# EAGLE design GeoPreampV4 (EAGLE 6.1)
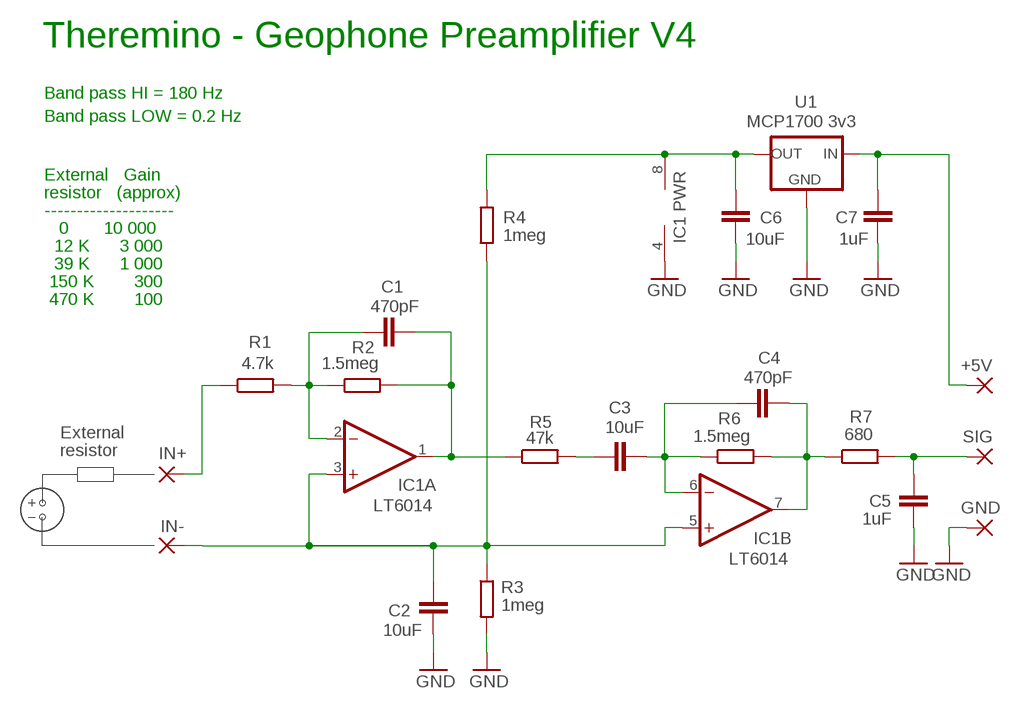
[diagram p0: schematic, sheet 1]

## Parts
+5V  WIREPADSMD1,27-2,54  [SMD1,27-2,54]
C1  470pF  C-EUC0805  [C0805]
C2  10uF  C-EUC0805  [C0805]
C3  10uF  C-EUC0805  [C0805]
C4  470pF  C-EUC0805  [C0805]
C5  1uF  C-EUC0805  [C0805]
C6  10uF  C-EUC0805  [C0805]
C7  1uF  C-EUC0805  [C0805]
GND  WIREPADSMD1,27-2,54  [SMD1,27-2,54]
IC1  LT6014  LMC6482D  [SOIC08_S]
IN+  WIREPADSMD1,27-2,54  [SMD1,27-2,54]
IN-  WIREPADSMD1,27-2,54  [SMD1,27-2,54]
R1  4.7k  R-EU_R0805  [R0805]
R2  1.5meg  R-EU_R0805  [R0805]
R3  1meg  R-EU_R1206  [R1206]
R4  1meg  R-EU_R1206_L  [R1206_L]
R5  47k  R-EU_R1206_L  [R1206_L]
R6  1.5meg  R-EU_R0805  [R0805]
R7  680  R-EU_R0805  [R0805]
SIG  WIREPADSMD1,27-2,54  [SMD1,27-2,54]
U1  MCP1700 3v3  MCP1700SOT23L  [SOT23_L]

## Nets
GND: C2.2 C5.1 C6.2 C7.2 GND.1(P) IC1.4(P:V-) R3.2 U1.1(GND)
N$1: C1.1 IC1.2(A:-IN) R1.2 R2.1
N$2: C3.1 C4.1 IC1.6(B:-IN) R6.1
N$3: C2.1 IC1.3(A:+IN) IC1.5(B:+IN) IN-.1(P) R3.1 R4.1
N$4: IN+.1(P) R1.1
N$5: C4.2 IC1.7(B:OUT) R6.2 R7.1
N$6: C1.2 IC1.1(A:OUT) R2.2 R5.1
N$7: C5.2 R7.2 SIG.1(P)
N$8: +5V.1(P) C7.1 U1.3(IN)
N$9: C3.2 R5.2
N$12: C6.1 IC1.8(P:V+) R4.2 U1.2(OUT)

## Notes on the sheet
- Theremino - Geophone Preamplifier V4
- Band pass HI = 180 Hz
- Band pass LOW = 0.2 Hz
- External   Gain
- resistor   (approx)
- --------------------
- 0       10 000
- IC1 PWR
- 12 K      3 000
- 39 K      1 000
- 150 K        300
- 470 K        100
- External
- resistor

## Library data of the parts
+5V GND IN+ IN- SIG = 00-LIVIO:WIREPAD: Wire PAD connect wire on PCB
C1-C7 = 00-LIVIO:C-EU: CAPACITOR, European symbol
IC1 = 00-LIVIO:LMC6482: OP AMP
R1-R7 = 00-LIVIO:R-EU_: RESISTOR, European symbol
U1 = 00-LIVIO:MCP1700: Linear regulator Quescient courrent 1.8uA Input 2.3v to 6v Output 1.2v 1.8v 2.5v 3.0v 3.3v 5.0v

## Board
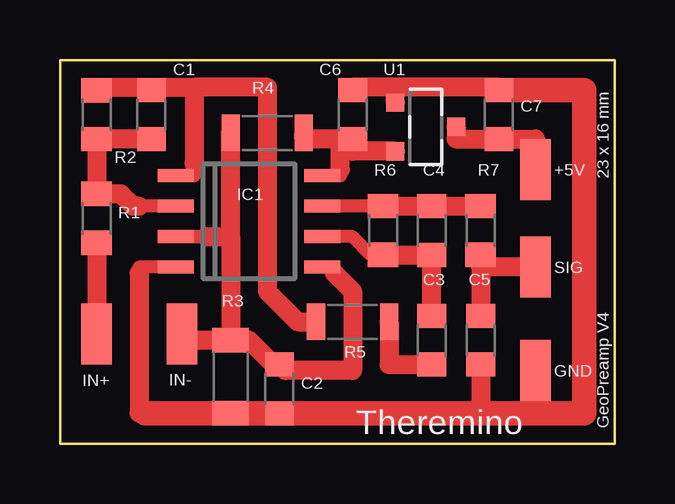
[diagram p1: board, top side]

Size 23.11 x 16 mm. Coordinates in mm from the lower left corner, seen from the top.
Outline: 23.11,0 0,0 0,16 23.11,16 23.11,0
Copper layers (1*16): Top 0.035mm / dielectric 1.5mm / Bottom 0.035mm
Design rules: minimum track width 10mil, minimum drill 27mil, track to track 27mil, track to pad 27mil, pad to pad 27mil, via to via 27mil, smd to smd 27mil, copper to edge 27mil, drill to drill 8mil, minimum pad ring 5mil, minimum via ring 8mil, stop-mask expansion 4mil, vias tented up to drill 0mil, thermal gap 41mil

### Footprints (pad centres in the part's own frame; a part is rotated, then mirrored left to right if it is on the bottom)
SMD1,27-2,54 = smd 1.27 x 2.54: 1 0,0
C0805 = smd 1 x 1.2: 1 -1.016,0; 2 1.016,0
SOIC08_S = smd 0.55 x 1.5: 1 -1.905,-3.048; 2 -0.635,-3.048; 3 0.635,-3.048; 4 1.905,-3.048; 5 1.905,3.048; 6 0.635,3.048; 7 -0.635,3.048; 8 -1.905,3.048
R0805 = smd 1.016 x 1.27: 1 -1.016,0; 2 1.016,0
R1206 = smd 1.016 x 1.524: 1 -1.524,0; 2 1.524,0
R1206_L = smd 0.762 x 1.524: 1 -1.524,0; 2 1.524,0
SOT23_L = smd 0.762 x 0.762: 1 -1.016,-1.27; 2 1.016,-1.27; 3 0,1.27

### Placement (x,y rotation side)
+5V  19.81,11.43 0 top
C1  3.81,13.72 90 top
C2  9.14,2.29 270 top
C3  15.49,4.32 270 top
C4  15.49,8.89 90 top
C5  17.53,4.32 90 top
C6  12.19,13.72 90 top
C7  18.29,13.72 90 top
GND  19.81,3.05 0 top
IC1  7.87,9.27 270 top
IN+  1.52,4.57 180 top
IN-  5.08,4.57 0 top
R1  1.52,9.4 90 top
R2  1.52,13.72 90 top
R3  7.11,2.79 270 top
R4  8.64,12.95 0 top
R5  12.19,5.08 0 top
R6  13.46,8.89 90 top
R7  17.53,8.89 270 top
SIG  19.81,7.37 0 top
U1  15.24,13.21 270 top

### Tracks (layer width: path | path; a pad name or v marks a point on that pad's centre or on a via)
GND
  Top 0.55: IC1.4 4.57,7.37 3.3,7.37 3.3,7.11
  Top 0.8: C7.2 18.29,14.86 13.97,14.86 | 13.97,14.86 12.19,14.86 C6.2 | 3.3,7.11 3.3,1.27 3.56,1.27 | U1.1 13.97,14.86 | C5.1 17.53,1.27 | GND.1 19.81,1.27
  Top 1.016: 3.56,1.27 R3.2 8.64,1.27 | 8.64,1.27 12.45,1.27 17.53,1.27 19.81,1.27 21.84,1.27 21.84,14.73 C7.2 | C2.2 8.64,1.27
N$1
  Top 0.55: IC1.2 3.3,9.91
  Top 0.8: 3.3,9.91 3.05,9.91 2.54,10.41 R1.2 R2.1 C1.1
N$2
  Top 0.55: R6.1 12.95,7.87 12.19,8.64 IC1.6
  Top 0.8: R6.1 C4.1 C3.1
N$3
  Top 0.55: 7.11,8.64 6.1,8.64 | 6.1,8.64 IC1.3 6.1,8.64 | IC1.5 11.43,7.37 11.43,7.11
  Top 0.8: 7.11,8.64 R4.1 | 11.43,7.11 12.19,6.35 12.19,3.05 9.4,3.05 C2.1 8.89,3.3 7.87,4.32 R3.1 | 6.1,8.64 7.11,8.64 | 7.11,8.64 R3.1 | IN-.1 5.08,4.32 R3.1
N$4
  Top 0.8: R1.1 IN+.1
N$5
  Top 0.55: R6.2 IC1.7
  Top 0.8: R6.2 C4.2 R7.1
N$6
  Top 0.55: IC1.1 5.59,11.18 5.59,11.68
  Top 0.8: R2.2 1.52,14.86 3.81,14.86 | 3.81,14.86 C1.2 3.81,14.86 | 3.81,14.86 5.59,14.86 | 5.59,14.86 5.59,11.68 | 5.59,14.86 5.84,14.86 8.64,14.86 8.64,11.43 8.64,6.35 9.91,5.08 R5.1
N$7
  Top 0.55: R7.2 17.53,7.37 R7.2
  Top 0.8: C5.2 17.53,7.37 SIG.1
N$8
  Top 0.8: +5V.1 19.81,12.7 C7.1 16.51,12.7 U1.3
N$9
  Top 0.8: R5.2 13.72,3.3 C3.2
N$12
  Top 0.55: IC1.8 11.68,11.18 11.68,11.43
  Top 0.8: 11.68,11.43 11.68,12.7 | 11.68,12.7 10.16,12.7 R4.2 | U1.2 12.19,12.19 C6.1 11.68,12.7

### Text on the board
tNames: 23 x 16 mm | GeoPreamp V4 | Theremino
